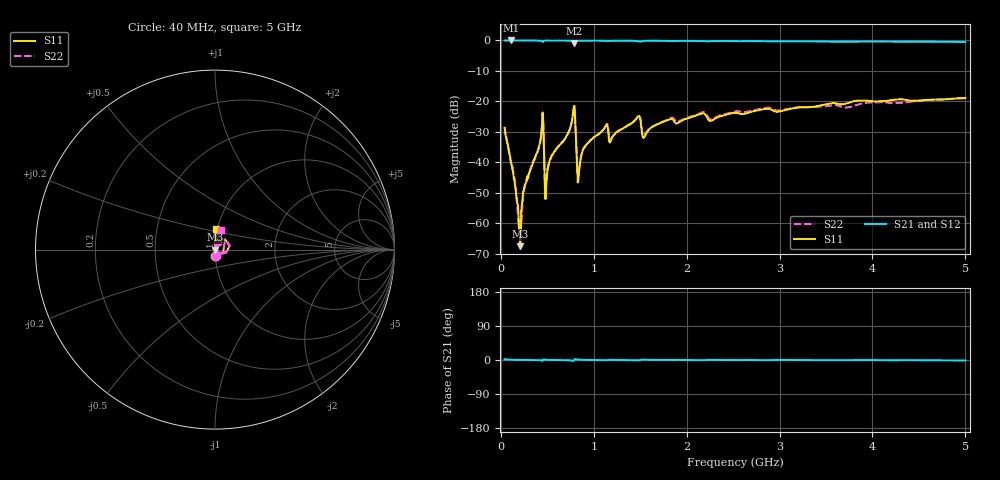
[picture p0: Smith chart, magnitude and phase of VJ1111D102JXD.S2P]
! VJ1111D102JXD
! DATE 02/15/2022  13:57
! CAPACITORS MOUNTED IN SERIES ON 25 MIL THICK MICROSTRIP SUBSTRATE
# GHz  S  MA  R  50.00
!  FREQ  S11M  S11A  S21M  S21A  S12M  S12A  S22M  S22A
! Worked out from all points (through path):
!   801 points, 40 MHz to 5 GHz, reference 50 ohm
!   highest |S21| = 0.00 dB at 108.2 MHz (marker M1); lowest = -0.8 dB at 790.2 MHz (marker M2)
!   lowest |S11| = -67.5 dB at 207.4 MHz (marker M3), VSWR 1.00, Z = 50 + j0.0381 ohm
!   |S11| at or under -10 dB: start of sweep to end of sweep
!   |S22| runs from -67.3 to -18.9 dB; largest |S21 - S12| = 0.012
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0.04  0.03682 -86.8  0.999 2.0  1 2.2  0.03802 -85.6
0.1082  0.01007 -92.3  1.001 0.7  0.9995 0.8  0.01003 -83.7
0.1454  0.005382 -83.6  0.9997 0.4  0.9976 0.5  0.005244 -92.4
0.1888  0.001473 -53.1  0.9997 0.3  0.9976 0.4  0.0009723 -62.1
0.2074  0.0004212 64.8  0.9993 0.3  1 0.2  0.0004323 19.2
0.2632  0.004419 82.1  0.9989 0.0  0.9985 0.1  0.004227 82.0
0.4306  0.02577 79.9  0.9918 -0.9  0.9986 -1.0  0.02607 80.8
0.4926  0.005349 81.8  0.9954 0.4  0.9992 0.5  0.005758 72.2
0.5484  0.01337 87.9  0.9947 -0.0  1.001 0.2  0.01265 85.1
0.7716  0.05572 69.6  0.9765 -2.0  0.9818 -2.0  0.0556 69.3
0.7902  0.08458 14.7  0.9144 -0.2  0.9185 -0.2  0.08472 15.3
0.8336  0.004935 48.6  0.9908 0.9  0.9974 0.9  0.006602 36.7
0.8708  0.01408 85.7  0.9936 0.5  0.9989 0.4  0.01388 80.4
1.125  0.03829 80.8  0.9885 -0.6  0.9923 -0.7  0.03884 78.6
1.187  0.02342 82.9  0.9902 0.3  0.9945 0.3  0.02465 73.7
1.4722  0.05592 75.7  0.976 -1.0  0.9833 -1.1  0.05651 70.6
1.5466  0.02639 78.2  0.9856 0.7  0.9892 0.6  0.02847 68.3
1.6954  0.04264 91.1  0.989 -0.0  0.9945 -0.1  0.04343 82.7
2.52  0.0649 88.7  0.9769 -0.3  0.9831 -0.4  0.06813 79.9
3.3508  0.08129 91.7  0.9651 -0.2  0.9711 -0.5  0.08046 79.0
4.1754  0.1032 88.8  0.9559 -0.7  0.9643 -0.9  0.09494 76.8
5  0.1135 87.9  0.9445 -1.3  0.9507 -1.5  0.1129 73.2
